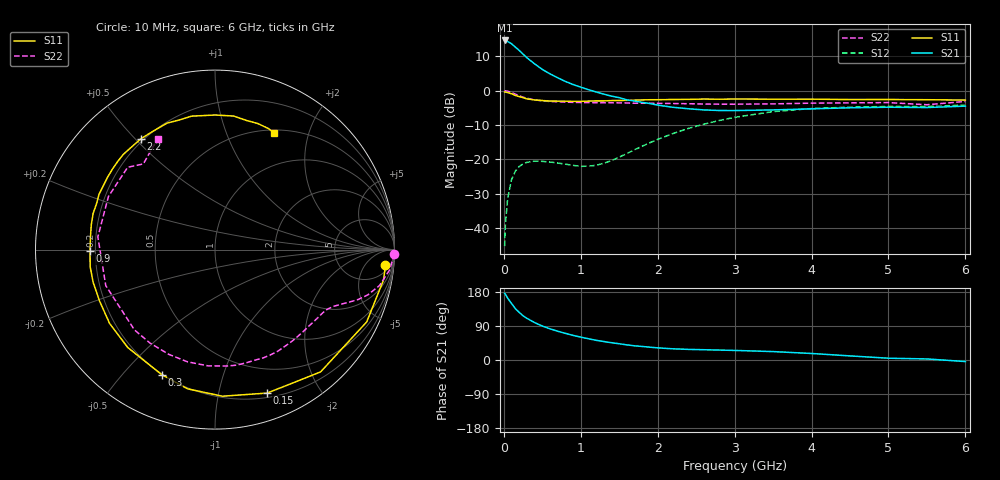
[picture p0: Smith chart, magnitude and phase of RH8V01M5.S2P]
! SIEMENS Small Signal Semiconductors
! BFR106
! Si NPN RF Bipolar Junction Transistor in SOT23
! VCE = 8 V  IC = 1.5 mA
! Common Emitter S-Parameters:  August  1996
# GHz  S  MA  R  50
!  f  S11  S21  S12  S22
! GHz  MAG  ANG  MAG  ANG  MAG  ANG  MAG  ANG
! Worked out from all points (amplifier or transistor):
!   36 points, 10 MHz to 6 GHz, reference 50 ohm
!   highest |S21| = 14.6 dB at 10 MHz (marker M1)
!   |S21| within 3 dB of that: start of sweep to 204.9 MHz
!   unconditionally stable (mu >= 1): 824.5 MHz to 1.815 GHz; 3.788 GHz to end of sweep
!   at 250 MHz: K = 0.29, MSG = 16.0 dB, |S12| = -21.4 dB
!   at 1.4 GHz: K = 1.29, MAG = 6.2 dB, |S12| = -20.4 dB
!   at 6 GHz: K = 1.02, MAG = -1.0 dB, |S12| = -4.2 dB
!   S11 on the Smith chart (normalised r, x): 10 MHz: 9, -17; 150 MHz: 0.24, -1.40; 300 MHz: 0.20, -0.64; 900 MHz: 0.18, -0.01; 2.2 GHz: 0.19, +0.52; 6 GHz: 0.54, +1.49
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0.01  0.9535 -5.3  5.385 176.0  0.0054 89.2  0.9999 -1.4
0.02  0.9542 -10.2  5.357 173.5  0.0111 86.1  0.9936 -2.7
0.05  0.9362 -25.5  5.195 163.0  0.027 75.9  0.9797 -6.6
0.1  0.9003 -49.2  4.822 149.2  0.0503 63.6  0.9385 -12.3
0.15  0.8506 -70.0  4.299 135.5  0.0672 52.7  0.8879 -16.5
0.2  0.8179 -87.1  3.859 125.7  0.0784 45.3  0.8433 -19.3
0.25  0.7906 -101.2  3.405 116.5  0.0855 38.9  0.8021 -21.4
0.3  0.7571 -113.1  3.012 109.9  0.09 34.8  0.7743 -22.9
0.4  0.7306 -131.7  2.455 98.8  0.094 28.4  0.7335 -25.5
0.5  0.717 -145.0  2.038 89.6  0.093 24.9  0.7088 -27.9
0.7  0.7029 -165.1  1.538 75.9  0.088 24.2  0.6872 -33.5
0.9  0.6962 -179.2  1.226 65.0  0.0814 30.4  0.6739 -39.6
1.1  0.7032 168.5  1.032 56.1  0.0791 43.0  0.668 -46.8
1.6  0.7221 145.8  0.734 39.9  0.121 72.6  0.6604 -66.1
2.2  0.7428 123.8  0.571 29.5  0.237 74.7  0.649 -93.3
2.8  0.7491 105.1  0.513 26.2  0.3667 62.3  0.6343 -124.8
3.5  0.7499 89.9  0.523 22.2  0.4938 44.4  0.6407 -161.7
4  0.7513 82.1  0.542 17.2  0.548 31.8  0.6565 173.8
4.5  0.7405 76.1  0.562 10.8  0.5743 20.8  0.6633 153.5
5  0.7419 71.2  0.573 4.7  0.5871 11.8  0.6687 136.7
5.5  0.7369 66.0  0.567 2.8  0.5857 7.4  0.6223 129.9
6  0.7278 63.0  0.594 -4.1  0.6156 -0.9  0.6954 117.4
